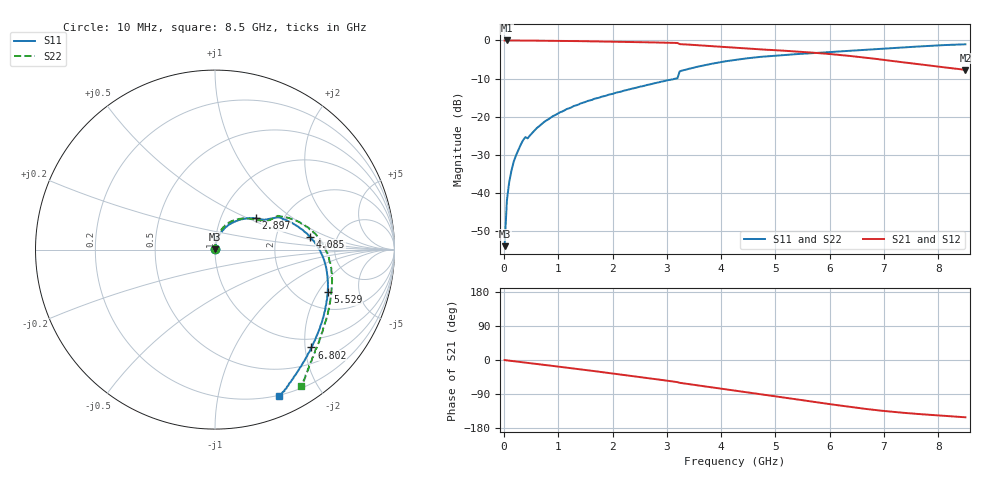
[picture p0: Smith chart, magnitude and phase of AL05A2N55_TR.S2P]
!AVX Corporation
!PN: AL05A2N55*TR
!Description: Air Core Inductor, 2.55nH, 3 Turns
!Agilent Technologies,E5071C,MY46102230,A.09.54
!Date: Mon Sep 03 16:13:44 2012
!Data & Calibration Information:
!Freq	S11:SOLT2(ON)	S21:SOLT2(ON)	S12:SOLT2(ON)	S22:SOLT2(ON)
# Hz S dB R 50
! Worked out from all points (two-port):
!   201 points, 10 MHz to 8.5 GHz, reference 50 ohm
!   highest |S21| = 0.00 dB at 52.45 MHz (marker M1); lowest = -7.7 dB at 8.5 GHz (marker M2)
!   |S21| within 3 dB of the highest: start of sweep to 5.495 GHz
!   lowest |S11| = -53.9 dB at 10 MHz (marker M3), VSWR 1.00, Z = 50 + j0.201 ohm
!   |S11| at or under -10 dB: start of sweep to 3.161 GHz
!   |S22| runs from -53.1 to -0.9 dB; largest |S21 - S12| = 0.015
!   S11 on the Smith chart (normalised r, x): 10 MHz: 1.00, +0.00; 2.897 GHz: 1.47, +0.56; 4.085 GHz: 3.15, +0.64; 5.529 GHz: 2.82, -2.44; 6.802 GHz: 0.81, -2.13; 8.5 GHz: 0.19, -1.51
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1e7  -53.92 87.8  -0.01 -0.2  -0.01 -1.1  -53.09 90.8
5.245e7  -41.90 87.4  -0.00 -1.0  0.04 -1.1  -41.81 87.7
9.49e7  -37.10 83.9  -0.01 -1.8  0.00 -1.8  -37.13 84.5
1.798e8  -31.68 82.9  -0.01 -3.3  0.00 -3.3  -31.65 84.5
3.0715e8  -27.32 80.2  -0.03 -5.5  -0.01 -5.6  -27.28 83.5
3.9205e8  -25.35 79.6  -0.04 -7.0  -0.03 -7.1  -25.29 81.5
4.345e8  -25.66 78.3  -0.04 -7.6  -0.03 -7.7  -25.67 81.0
6.043e8  -22.95 75.4  -0.06 -10.6  -0.05 -10.6  -22.98 78.3
9.0145e8  -19.82 71.0  -0.10 -15.7  -0.09 -15.8  -19.89 73.9
1.4533e9  -16.34 62.2  -0.19 -25.5  -0.18 -25.6  -16.36 65.5
2.85415e9  -10.96 38.0  -0.55 -51.6  -0.55 -51.7  -10.92 36.0
2.8966e9  -10.80 37.4  -0.56 -52.5  -0.56 -52.5  -10.82 34.8
3.19375e9  -9.92 31.3  -0.67 -58.4  -0.66 -58.4  -9.92 28.4
3.2362e9  -8.10 27.2  -0.96 -60.2  -0.95 -60.2  -8.01 28.2
4.0852e9  -5.45 7.8  -1.73 -77.4  -1.73 -77.4  -5.41 13.0
4.255e9  -5.10 4.3  -1.90 -80.8  -1.90 -80.9  -5.10 9.9
4.89175e9  -4.10 -8.4  -2.46 -93.6  -2.47 -93.6  -4.08 -1.6
5.5285e9  -3.45 -20.7  -3.04 -106.7  -3.04 -106.8  -3.43 -14.4
5.6983e9  -3.31 -24.0  -3.22 -110.3  -3.21 -110.3  -3.29 -18.2
6.802e9  -2.32 -45.4  -4.75 -131.4  -4.75 -131.4  -2.27 -40.9
7.09915e9  -2.05 -50.5  -5.26 -135.9  -5.27 -136.0  -1.97 -45.7
8.5e9  -1.01 -66.3  -7.70 -151.2  -7.70 -151.2  -0.93 -57.9
